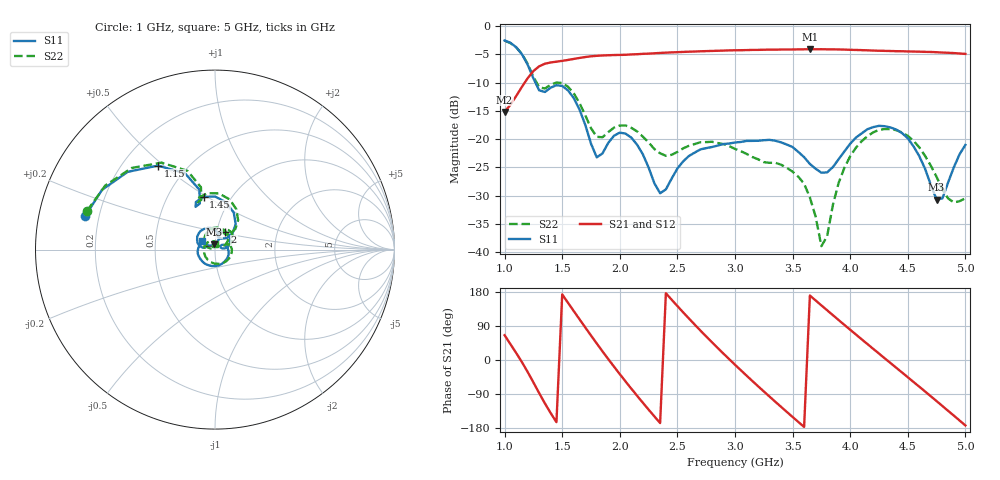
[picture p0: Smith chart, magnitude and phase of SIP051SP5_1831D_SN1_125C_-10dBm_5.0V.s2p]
# GHz  S  dB  R  50
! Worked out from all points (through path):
!   81 points, 1 GHz to 5 GHz, reference 50 ohm
!   highest |S21| = -4.08 dB at 3.65 GHz (marker M1); lowest = -15.2 dB at 1 GHz (marker M2)
!   lowest |S11| = -30.7 dB at 4.75 GHz (marker M3), VSWR 1.06, Z = 49.4 + j2.85 ohm
!   |S11| at or under -10 dB: 1.268 GHz to end of sweep
!   |S22| runs from -38.9 to -2.6 dB; largest |S21 - S12| = 0.0018
!   S11 on the Smith chart (normalised r, x): 1 GHz: 0.15, +0.12; 1.15 GHz: 0.35, +0.48; 1.45 GHz: 0.75, +0.48; 2 GHz: 1.10, +0.22; 5 GHz: 0.86, +0.08
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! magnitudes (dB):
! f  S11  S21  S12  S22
! 1 GHz  -2.5  -15.2  -15.2  -2.6
! 1.15 GHz  -4.9  -10.7  -10.7  -4.9
! 1.3 GHz  -11.4  -7.1  -7.1  -10.8
! 1.45 GHz  -10.4  -6.3  -6.3  -10.0
! 1.6 GHz  -12.7  -5.8  -5.8  -11.9
! 1.7 GHz  -17.4  -5.5  -5.5  -15.8
! 1.8 GHz  -23.2  -5.2  -5.2  -19.6
! 2 GHz  -18.8  -5.1  -5.1  -17.6
! 2.15 GHz  -21.0  -5.0  -5.0  -18.6
! 2.35 GHz  -29.6  -4.7  -4.7  -22.5
! 2.6 GHz  -23.0  -4.5  -4.5  -21.2
! 3 GHz  -20.6  -4.3  -4.3  -21.7
! 3.5 GHz  -21.4  -4.1  -4.1  -25.7
! 3.65 GHz  -24.4  -4.1  -4.1  -30.3
! 3.7 GHz  -25.2  -4.1  -4.1  -33.7
! 3.75 GHz  -25.9  -4.1  -4.1  -38.9
! 4 GHz  -20.8  -4.2  -4.2  -23.0
! 4.35 GHz  -17.9  -4.4  -4.4  -18.2
! 4.55 GHz  -21.3  -4.5  -4.5  -20.3
! 4.75 GHz  -30.7  -4.6  -4.6  -26.7
! 4.85 GHz  -27.6  -4.7  -4.7  -30.5
! 5 GHz  -21.0  -4.9  -4.9  -30.4
